(* Logix 5000 AddOnInstructionDefinition export EH_Dosimag_IOL; software revision 38.00 *)

TYPE EH_CommAOI_Data :
STRUCT
   Device_Comm_Error : BOOL;
   CommSuccess : BOOL;
   CommFailed : BOOL;
   CommTimeOut : BOOL;
   StateDone : BOOL;
   NewState : BOOL;
   OldState : SINT;
   PortSize : SINT;
   DevicePort : SINT;
   MaxState : SINT;
   State : SINT;
   VendorID : INT;
   DeviceID : DINT;
   CyclicData : INT[16];
   AcyclicData : DINT[8];
   ReplayIndex : INT;
   AOI_Diagnostic : DINT;
   ConnectionStatus : DINT;
   OutputData : INT[16];
END_STRUCT
END_TYPE

ADD_ON_INSTRUCTION EH_Dosimag_IOL   (* revision 1.1, vendor Endress+Hauser *)
// Dosimag D5AB Rev 1 IO-Link
// Revision note:
// 1.1 Changed the Datatype from Unsigned to Signed
// ZeroPoint adjustment update
// Add Disconnect check
// Add condition PulseSimulation
VAR_IN_OUT
   DataToSend : INT[10]; {required}
   CommAOIBusy : DINT; {required}
   ActiveComPort : DINT; {required}
   DeviceAOISendRequest : DINT; {required}
   CommError : INT; {required}
   DeviceData : EH_CommAOI_Data; {required}
END_VAR
VAR_INPUT
   iSetPulseSimulation : BOOL; {visible}
   iSimulationOnOff : BOOL; {access None, visible}
   iAmountPulses : INT; {visible}
   iSetTotalizerPresetValue : BOOL; {visible}
   iTotalizer1PresetValue : REAL; {visible}
   iTotalizer_Hold : BOOL; {visible}
   iTotalizer_ResetTotalize : BOOL; {visible}
   iTotalizer_ResetHold : BOOL; {visible}
   iTotalizer_Totalize : BOOL; {visible}
   iParameterize : BOOL; {visible}
   iFlowDamping : REAL; {visible}
   iPressureShockSupression : REAL; {visible}
   iIntegrationTime : REAL; {visible}
   iMeasuringPeriod : REAL; {visible}
   iLowFlowCutoffValue : REAL; {visible}
   iFlowOverride : BOOL; {visible}
   iStartZeroPointAdjustment : BOOL; {visible}
END_VAR
VAR_OUTPUT
   qVendor_ID : DINT; {access Read Only, visible}
   qDevice_ID : DINT; {access Read Only, visible}
   qVolumeFlow : REAL; {visible}
   qTemperature : REAL; {visible}
   qTotalizer1 : REAL; {access Read Only, visible}
   qExtendedDeviceStatus : INT; {access Read Only, visible}
   qZeroPointStatus : SINT; {access Read Only, visible}
   qReadProgress : SINT; {access Read Only, visible}
   qSSC1_1 : BOOL; {access Read Only, visible}
   qSSC1_2 : BOOL; {access Read Only, visible}
   qSSC2_1 : BOOL; {access Read Only, visible}
   qSSC2_2 : BOOL; {access Read Only, visible}
   qSSC3_1 : BOOL; {access Read Only, visible}
   qSSC3_2 : BOOL; {access Read Only, visible}
   qSSC4_1 : BOOL; {access Read Only, visible}
   qSSC4_2 : BOOL; {access Read Only, visible}
   qAOI_Diagnostic : DINT; {access Read Only, visible}
END_VAR
VAR_IN_OUT
   qAOI_Diagnostic_String : STRING; {required}
END_VAR
VAR_OUTPUT
   qActual_Diagnostics_Code : DINT; {access Read Only, visible}
END_VAR
VAR_IN_OUT
   qActual_Diagnostics_String : STRING; {required}
END_VAR
VAR_OUTPUT
   qLast_Diagnostics_Code : DINT; {visible}
END_VAR
VAR_IN_OUT
   qLast_Diagnostics_String : STRING; {required}
END_VAR
VAR_OUTPUT
   qCommError : DINT; {access None}
   qCommunicationBusy : DINT; {access Read Only, visible}
   qDeviceConnectionError : BOOL; {access Read Only, visible}
END_VAR
VAR
   Temp_DINT : DINT; {access None}
   CMD_Index : INT; {access None}
   CMD_Subindex : INT; {access None}
   CMD_ByteLength : INT; {access None}
   oldCondStatus : INT; {access None}
   SetSimulation : SINT; {access None}
   SetTotalizer : SINT; {access None}
   oldSetTotalizer : SINT; {access None}
   oldStartZeroPointAdjustment : SINT; {access None}
   Trigger : BOOL; {access None}
   CMD_Rd : BOOL; {access None}
   CMD_Wr : BOOL; {access None}
   SimulationDINT : DINT; {access None}
   AOI_Prio : BOOL; {access None}
   StateMin : DINT; {access None}
   firstTimeDone : BOOL; {access None}
   CondStatusChanged : BOOL; {access None}
   Calc_MassFlow : DINT; {access None}
   Calc_Temperature : DINT; {access None}
   Calc_Totalizer1 : DINT; {access None}
   Calc_ExtendedDeviceStatus : DINT; {access None}
   CondStatusActive : BOOL; {access None}
   ActiveAOI : BOOL; {access None}
   TotActive : BOOL; {access None}
   Skip : BOOL; {access None}
   StartZeroPointAdjustment : SINT; {access None}
   Parameterize : SINT; {access None}
   oldParameterize : SINT; {access None}
   oldSetPulseSimulation : SINT; {access None}
   TotChanged : BOOL; {access None}
   DeviceID : DINT; {access None}
   SetPulseSimulation : SINT; {access None}
   zeroPointStatus : SINT; {access None}
   StartZeroPointAdjustmentChanged : BOOL; {access None}
   ParameterizeChanged : BOOL; {access None}
   PulseSimChanged : BOOL; {access None}
   TRUE : BOOL := 1; {access None}
   FALSE : BOOL; {access None}
   ParameterizeActive : BOOL; {access None}
   PulseSimActive : BOOL; {access None}
   ZeroPointActive : BOOL; {access None}
   StandardTimer : FBD_TIMER; {access None}
   temp_string1 : STRING; {access None}
   temp_string2 : STRING; {access None}
   Calc_VolumeFLow : DINT; {access None}
   IntegrationTimeREAL : REAL; {access None}
   MeasuringPeriodREAL : REAL; {access None}
   onlyonce : BOOL; {access None}
END_VAR

ROUTINE Logic   (* structured text *)
// Picomag Communication via AL1323
   // =======================================================================
   // Endress+Hauser Digital Solutions
   // ©Copyright (2024) All Rights Reserved
   // =======================================================================
   // Name:                EH_Dosimag_IOL
   // Version:             1.1
   // Datum:               02.2026
   // Library:             01.01.00
   // Engineering:         Studio5000 V38.00.00
   // Author:              EH
   // =======================================================================
   
   qAOI_Diagnostic := DeviceData.AOI_Diagnostic;
   qCommunicationBusy := CommAOIBusy;
   DeviceID := 9729281;
   StateMin := 0;
   DeviceData.MaxState := 98;
   
   if DeviceData.DevicePort = 0 or DeviceData.DeviceID <> DeviceID or DeviceData.ConnectionStatus <> 1 then
   
   	qVendor_ID := DeviceData.VendorID;
   	qDevice_ID := DeviceData.DeviceID;
   	qVolumeFlow := 0;
   	qTemperature := 0;
   	qTotalizer1	:= 0;
   	qExtendedDeviceStatus := 0;
   	qSSC1_1	:= FALSE;
   	qSSC1_2	:= FALSE;
   	qSSC2_1	:= FALSE;
   	qSSC2_2	:= FALSE;
   	qSSC3_1	:= FALSE;
   	qSSC3_2	:= FALSE;
   	qSSC4_1	:= FALSE;
   	qSSC4_2	:= FALSE;
   	qActual_Diagnostics_Code := 0;
   	qActual_Diagnostics_String := '';
   	qLast_Diagnostics_Code := 0;
   	qLast_Diagnostics_String := '';
   	qReadProgress := 0;
   	qZeroPointStatus := 0;
   	oldCondStatus := 0;
   	CondStatusChanged := FALSE;
   	zeroPointStatus := 0;
   
   	if DeviceData.DevicePort = 0 then
   
   		qAOI_Diagnostic_String	:= 'Device Port is Zero';
   		DeviceData.AOI_Diagnostic.1 := TRUE;
   
   	elsif DeviceData.ConnectionStatus <> 1 then
   
   		qAOI_Diagnostic_String	:= 'No Device connected';
   		qDeviceConnectionError := TRUE;
   
   	elsif DeviceData.DeviceID <> DeviceID then
   
   		qAOI_Diagnostic_String	:= 'Wrong DeviceID';
   		DeviceData.AOI_Diagnostic.2 := TRUE;
   	end_if;
   
   else
   
   	if qActual_Diagnostics_Code = 0  then
   
   		qActual_Diagnostics_String	:= '--------';
   
   	end_if;
   
   	if qLast_Diagnostics_Code = 0 then
   
   		qLast_Diagnostics_String	:= '--------';
   
   	end_if;
   
   	qAOI_Diagnostic_String := '';
   	DeviceData.AOI_Diagnostic.1 := FALSE;
   	qDeviceConnectionError := FALSE;
   	DeviceData.AOI_Diagnostic.2  := FALSE;
   
   end_if;
   
   // Case device disconnected during communication to avoid blocking the communication
   if (DeviceData.AOI_Diagnostic.0 or qDeviceConnectionError or DeviceData.AOI_Diagnostic.2) and ActiveAOI and ActiveComPort = DeviceData.DevicePort and CommAOIBusy = 1 then
   
   	DeviceData.State := 0;
   	CommAOIBusy := 0;
   	DeviceAOISendRequest.[DeviceData.DevicePort] := 0;
   	ActiveComPort := 0;
   	ActiveAOI := 0;
   	DataToSend[0] := 0;
   	DataToSend[1] := 0;
   	DataToSend[2] := 0;
   	DataToSend[3] := 0;
   	DataToSend[4] := 0;
   	DataToSend[5] := 0;
   	DataToSend[6] := 0;
   	DataToSend[7] := 0;
   	DataToSend[8] := 0;
   	DataToSend[9] := 0;
   	DeviceData.StateDone := FALSE;
   	DeviceData.NewState := FALSE;
   	DeviceData.OldState := 0;
   	ActiveAOI := FALSE;
   
   end_if;
   
   if not DeviceData.AOI_Diagnostic.0
   	and not qDeviceConnectionError
   	and not DeviceData.AOI_Diagnostic.2
   	and DeviceData.DevicePort > 0 then
   
   	//*********************************
   	//Vendor ID
   	//*********************************
   
   		qVendor_ID := DeviceData.VendorID;
   
   	//*********************************
   	//Device ID
   	//*********************************
   
   		qDevice_ID := DeviceData.DeviceID;
   
   	//*********************************
   	// Dosimag
   	//*********************************
   
   		Calc_VolumeFLow			    := 0;
   		// Offset +2 is not used
   		Calc_Temperature			:= 4;
   		Calc_Totalizer1				:= 6;
   		Calc_ExtendedDeviceStatus	:= 8;
   
   	//*********************************
   	//Process VolumeFlow
   	//*********************************
   
   		Temp_DINT	 := DeviceData.CyclicData[Calc_VolumeFLow+1];
   		Temp_DINT.8	 := DeviceData.CyclicData[Calc_VolumeFLow+1].8;
   		Temp_DINT.9  := DeviceData.CyclicData[Calc_VolumeFLow+1].9;
   		Temp_DINT.10 := DeviceData.CyclicData[Calc_VolumeFLow+1].10;
   		Temp_DINT.11 := DeviceData.CyclicData[Calc_VolumeFLow+1].11;
   		Temp_DINT.12 := DeviceData.CyclicData[Calc_VolumeFLow+1].12;
   		Temp_DINT.13 := DeviceData.CyclicData[Calc_VolumeFLow+1].13;
   		Temp_DINT.14 := DeviceData.CyclicData[Calc_VolumeFLow+1].14;
   		Temp_DINT.15 := DeviceData.CyclicData[Calc_VolumeFLow+1].15;
   		Temp_DINT.16 := DeviceData.CyclicData[Calc_VolumeFLow].0;
   		Temp_DINT.17 := DeviceData.CyclicData[Calc_VolumeFLow].1;
   		Temp_DINT.18 := DeviceData.CyclicData[Calc_VolumeFLow].2;
   		Temp_DINT.19 := DeviceData.CyclicData[Calc_VolumeFLow].3;
   		Temp_DINT.20 := DeviceData.CyclicData[Calc_VolumeFLow].4;
   		Temp_DINT.21 := DeviceData.CyclicData[Calc_VolumeFLow].5;
   		Temp_DINT.22 := DeviceData.CyclicData[Calc_VolumeFLow].6;
   		Temp_DINT.23 := DeviceData.CyclicData[Calc_VolumeFLow].7;
   		Temp_DINT.24 := DeviceData.CyclicData[Calc_VolumeFLow].8;
   		Temp_DINT.25 := DeviceData.CyclicData[Calc_VolumeFLow].9;
   		Temp_DINT.26 := DeviceData.CyclicData[Calc_VolumeFLow].10;
   		Temp_DINT.27 := DeviceData.CyclicData[Calc_VolumeFLow].11;
   		Temp_DINT.28 := DeviceData.CyclicData[Calc_VolumeFLow].12;
   		Temp_DINT.29 := DeviceData.CyclicData[Calc_VolumeFLow].13;
   		Temp_DINT.30 := DeviceData.CyclicData[Calc_VolumeFLow].14;
   		Temp_DINT.31 := DeviceData.CyclicData[Calc_VolumeFLow].15;
   
   		COP(Temp_DINT,qVolumeFlow,1);
   
   
   	//*********************************
   	//Process Data Temperature
   	//*********************************
   
   		Temp_DINT	 := DeviceData.CyclicData[Calc_Temperature+1];
   		Temp_DINT.8	 := DeviceData.CyclicData[Calc_Temperature+1].8;
   		Temp_DINT.9	 := DeviceData.CyclicData[Calc_Temperature+1].9;
   		Temp_DINT.10 := DeviceData.CyclicData[Calc_Temperature+1].10;
   		Temp_DINT.11 := DeviceData.CyclicData[Calc_Temperature+1].11;
   		Temp_DINT.12 := DeviceData.CyclicData[Calc_Temperature+1].12;
   		Temp_DINT.13 := DeviceData.CyclicData[Calc_Temperature+1].13;
   		Temp_DINT.14 := DeviceData.CyclicData[Calc_Temperature+1].14;
   		Temp_DINT.15 := DeviceData.CyclicData[Calc_Temperature+1].15;
   		Temp_DINT.16 := DeviceData.CyclicData[Calc_Temperature].0;
   		Temp_DINT.17 := DeviceData.CyclicData[Calc_Temperature].1;
   		Temp_DINT.18 := DeviceData.CyclicData[Calc_Temperature].2;
   		Temp_DINT.19 := DeviceData.CyclicData[Calc_Temperature].3;
   		Temp_DINT.20 := DeviceData.CyclicData[Calc_Temperature].4;
   		Temp_DINT.21 := DeviceData.CyclicData[Calc_Temperature].5;
   		Temp_DINT.22 := DeviceData.CyclicData[Calc_Temperature].6;
   		Temp_DINT.23 := DeviceData.CyclicData[Calc_Temperature].7;
   		Temp_DINT.24 := DeviceData.CyclicData[Calc_Temperature].8;
   		Temp_DINT.25 := DeviceData.CyclicData[Calc_Temperature].9;
   		Temp_DINT.26 := DeviceData.CyclicData[Calc_Temperature].10;
   		Temp_DINT.27 := DeviceData.CyclicData[Calc_Temperature].11;
   		Temp_DINT.28 := DeviceData.CyclicData[Calc_Temperature].12;
   		Temp_DINT.29 := DeviceData.CyclicData[Calc_Temperature].13;
   		Temp_DINT.30 := DeviceData.CyclicData[Calc_Temperature].14;
   		Temp_DINT.31 := DeviceData.CyclicData[Calc_Temperature].15;
   
   		COP(Temp_DINT,qTemperature,1);
   
   	//*********************************
   	// Process Parameter Totalizer1
   	//*********************************
   
   		Temp_DINT	 := DeviceData.CyclicData[Calc_Totalizer1+1];
   		Temp_DINT.8  := DeviceData.CyclicData[Calc_Totalizer1+1].8;
   		Temp_DINT.9  := DeviceData.CyclicData[Calc_Totalizer1+1].9;
   		Temp_DINT.10 := DeviceData.CyclicData[Calc_Totalizer1+1].10;
   		Temp_DINT.11 := DeviceData.CyclicData[Calc_Totalizer1+1].11;
   		Temp_DINT.12 := DeviceData.CyclicData[Calc_Totalizer1+1].12;
   		Temp_DINT.13 := DeviceData.CyclicData[Calc_Totalizer1+1].13;
   		Temp_DINT.14 := DeviceData.CyclicData[Calc_Totalizer1+1].14;
   		Temp_DINT.15 := DeviceData.CyclicData[Calc_Totalizer1+1].15;
   		Temp_DINT.16 := DeviceData.CyclicData[Calc_Totalizer1].0;
   		Temp_DINT.17 := DeviceData.CyclicData[Calc_Totalizer1].1;
   		Temp_DINT.18 := DeviceData.CyclicData[Calc_Totalizer1].2;
   		Temp_DINT.19 := DeviceData.CyclicData[Calc_Totalizer1].3;
   		Temp_DINT.20 := DeviceData.CyclicData[Calc_Totalizer1].4;
   		Temp_DINT.21 := DeviceData.CyclicData[Calc_Totalizer1].5;
   		Temp_DINT.22 := DeviceData.CyclicData[Calc_Totalizer1].6;
   		Temp_DINT.23 := DeviceData.CyclicData[Calc_Totalizer1].7;
   		Temp_DINT.24 := DeviceData.CyclicData[Calc_Totalizer1].8;
   		Temp_DINT.25 := DeviceData.CyclicData[Calc_Totalizer1].9;
   		Temp_DINT.26 := DeviceData.CyclicData[Calc_Totalizer1].10;
   		Temp_DINT.27 := DeviceData.CyclicData[Calc_Totalizer1].11;
   		Temp_DINT.28 := DeviceData.CyclicData[Calc_Totalizer1].12;
   		Temp_DINT.29 := DeviceData.CyclicData[Calc_Totalizer1].13;
   		Temp_DINT.30 := DeviceData.CyclicData[Calc_Totalizer1].14;
   		Temp_DINT.31 := DeviceData.CyclicData[Calc_Totalizer1].15;
   
   		COP(Temp_DINT,qTotalizer1,1);
   
   	//*********************************
   	// Extended device Status
   	//*********************************
   
   		qExtendedDeviceStatus.0 := DeviceData.CyclicData[Calc_ExtendedDeviceStatus].8;
   		qExtendedDeviceStatus.1 := DeviceData.CyclicData[Calc_ExtendedDeviceStatus].9;
   		qExtendedDeviceStatus.2 := DeviceData.CyclicData[Calc_ExtendedDeviceStatus].10;
   		qExtendedDeviceStatus.3 := DeviceData.CyclicData[Calc_ExtendedDeviceStatus].11;
   		qExtendedDeviceStatus.4 := DeviceData.CyclicData[Calc_ExtendedDeviceStatus].12;
   		qExtendedDeviceStatus.5 := DeviceData.CyclicData[Calc_ExtendedDeviceStatus].13;
   		qExtendedDeviceStatus.6 := DeviceData.CyclicData[Calc_ExtendedDeviceStatus].14;
   		qExtendedDeviceStatus.7 := DeviceData.CyclicData[Calc_ExtendedDeviceStatus].15;
   
   	//*********************************
   	// Process Parameter SSC
   	//*********************************
   
   		qSSC1_1 := DeviceData.CyclicData[Calc_ExtendedDeviceStatus].0;
   		qSSC1_2 := DeviceData.CyclicData[Calc_ExtendedDeviceStatus].1;
   
   		qSSC2_1 := DeviceData.CyclicData[Calc_ExtendedDeviceStatus].2;
   		qSSC2_2 := DeviceData.CyclicData[Calc_ExtendedDeviceStatus].3;
   
   		qSSC3_1 := DeviceData.CyclicData[Calc_ExtendedDeviceStatus].4;
   		qSSC3_2 := DeviceData.CyclicData[Calc_ExtendedDeviceStatus].5;
   
   		qSSC4_1 := DeviceData.CyclicData[Calc_ExtendedDeviceStatus].6;
   		qSSC4_2 := DeviceData.CyclicData[Calc_ExtendedDeviceStatus].7;
   
   	//*********************************
   	// Process Output Parameter
   	//*********************************
   
   		//DeviceData.OutputData[0].4 := iDeviceSearch;		//Device Specific
   		DeviceData.OutputData[0].5 := iFlowOverride;
   		DeviceData.OutputData[0].6 := iTotalizer_Hold;
   		DeviceData.OutputData[0].7 := iTotalizer_ResetTotalize;
   		DeviceData.OutputData[0].8 := iTotalizer_ResetHold;
   		DeviceData.OutputData[0].9 := iTotalizer_Totalize;
   
   	//*********************************
   	// Checking for Changed Status
   	//*********************************
   
   		SetPulseSimulation.0 := iSetPulseSimulation;
   		SetTotalizer.0 := iSetTotalizerPresetValue;
   		Parameterize.0 := iParameterize;
   		StartZeroPointAdjustment.0 := iStartZeroPointAdjustment;
   
   		if oldCondStatus <> qExtendedDeviceStatus and not CondStatusChanged then
   
   			CondStatusChanged := TRUE;
   			oldCondStatus := qExtendedDeviceStatus;
   
   		end_if;
   
   		if oldSetPulseSimulation <> SetPulseSimulation and not PulseSimChanged then
   
   			if oldSetPulseSimulation < SetPulseSimulation then
   
   				PulseSimChanged := TRUE;
   
   			end_if;
   
   			oldSetPulseSimulation := SetPulseSimulation;
   
   		end_if;
   
   		if oldStartZeroPointAdjustment <> StartZeroPointAdjustment and not StartZeroPointAdjustmentChanged then
   
   			if oldStartZeroPointAdjustment < StartZeroPointAdjustment then
   
   				StartZeroPointAdjustmentChanged := TRUE;
   
   			end_if;
   
   			oldStartZeroPointAdjustment := StartZeroPointAdjustment;
   
   		end_if;
   
   		if oldParameterize <> Parameterize and not ParameterizeChanged then
   
   			if oldParameterize < Parameterize then
   
   				ParameterizeChanged := TRUE;
   
   			end_if;
   
   			oldParameterize := Parameterize;
   
   		end_if;
   
   		if oldSetTotalizer <> SetTotalizer and not TotChanged then
   
   			if oldSetTotalizer < SetTotalizer then
   
   				TotChanged := TRUE;
   
   			end_if;
   
   			oldSetTotalizer := SetTotalizer;
   
   		end_if;
   
   		if CondStatusChanged
   		and not ActiveAOI
   		and not CondStatusActive
   		and not Skip then
   
   			DeviceAOISendRequest.[DeviceData.DevicePort] := TRUE;
   			CondStatusActive := TRUE;
   			Skip := TRUE;
   
   		elsif PulseSimChanged
   			and not ActiveAOI
   			and not PulseSimActive
   			and not Skip then
   
   			DeviceAOISendRequest.[DeviceData.DevicePort] := TRUE;
   			PulseSimActive := TRUE;
   			Skip := TRUE;
   
   		elsif TotChanged
   			and not ActiveAOI
   			and not TotActive
   			and not Skip then
   
   			DeviceAOISendRequest.[DeviceData.DevicePort] := TRUE;
   			TotActive := TRUE;
   			Skip := TRUE;
   
   		elsif StartZeroPointAdjustmentChanged
   			and not ActiveAOI
   			and not ZeroPointActive
   			and not Skip then
   
   			DeviceAOISendRequest.[DeviceData.DevicePort] := TRUE;
   			ZeroPointActive := TRUE;
   			Skip := TRUE;
   
   		elsif ParameterizeChanged
   			and not ActiveAOI
   			and not ParameterizeActive
   			and not Skip then
   
   			DeviceAOISendRequest.[DeviceData.DevicePort] := TRUE;
   			ParameterizeActive := TRUE;
   			Skip := TRUE;
   
   		end_if;
   
   		if ActiveComPort = DeviceData.DevicePort then
   
   			AOI_Prio :=TRUE;
   
   		else
   
   			AOI_Prio := FALSE;
   
   		end_if;
   
   		if (PulseSimActive or TotActive or CondStatusActive or ParameterizeActive or ZeroPointActive) and CommAOIBusy = 1  and DeviceData.State = 0 and AOI_Prio and not ActiveAOI then
   
   			ActiveAOI := TRUE;
   			Skip := FALSE;
   
   		end_if;
   
   		qCommunicationBusy := CommAOIBusy;
   		qAOI_Diagnostic :=DeviceData.AOI_Diagnostic;
   
   	//*********************************
   	// States for Execution
   	//*********************************
   
   	if ActiveAOI or DeviceData.State = DeviceData.MaxState then
   
   	case DeviceData.State of
   
   		//*********************************
   		0: // Idle
   		//*********************************
   
   			// Initializing
   			Trigger := FALSE;
   			CMD_Index := 0;
   			CMD_Subindex := 0;
   			CMD_Wr := FALSE;
   			CMD_Rd := FALSE;
   		    CMD_ByteLength := 0;
   
   			if DeviceData.DevicePort = ActiveComPort then
   					DeviceData.CommSuccess := FALSE;
   					DeviceData.CommTimeOut := FALSE;
   					DeviceData.NewState := TRUE;
   					DeviceData.StateDone := FALSE;
   			end_if;
   
   			// Wait for trigger
   			if ParameterizeActive then
   
   				DeviceData.AOI_Diagnostic := 0;
   				DeviceData.State := 6;
   
   			elsif PulseSimActive then
   
   				DeviceData.AOI_Diagnostic := 0;
   				DeviceData.State := 15;
   
   			elsif TotActive then
   				DeviceData.AOI_Diagnostic := 0;
   				DeviceData.State := 20;
   
   			elsif ZeroPointActive then
   
   				DeviceData.AOI_Diagnostic := 0;
   				qReadProgress := 0;
   				qZeroPointStatus := 0;
   				DeviceData.State := 30;
   
   			elsif CondStatusChanged then
   
   				DeviceData.State := 90;
   
   			end_if;
   
   		//*********************************
   		6: // Set Flow Damping
   		//*********************************
   
   			CMD_Index := 8550;
   			CMD_Subindex := 0;
   			CMD_Wr := TRUE;
   			CMD_Rd := FALSE;
   			CMD_ByteLength := 4;
   			DataToSend[6]:= 0;
   			DataToSend[7]:= 0;
   
   			// Time in seconds
   			COP(iFlowDamping,SimulationDINT,1);		// Copy the Bits from the Real in a DINT
   
   			DataToSend[6].0 :=  SimulationDINT.24;
   			DataToSend[6].1 :=  SimulationDINT.25;
   			DataToSend[6].2 :=  SimulationDINT.26;
   			DataToSend[6].3 :=  SimulationDINT.27;
   			DataToSend[6].4 :=  SimulationDINT.28;
   			DataToSend[6].5 :=  SimulationDINT.29;
   			DataToSend[6].6 :=  SimulationDINT.30;
   			DataToSend[6].7 :=  SimulationDINT.31;
   			DataToSend[6].8 :=  SimulationDINT.16;
   			DataToSend[6].9 :=  SimulationDINT.17;
   			DataToSend[6].10 := SimulationDINT.18;
   			DataToSend[6].11 := SimulationDINT.19;
   			DataToSend[6].12 := SimulationDINT.20;
   			DataToSend[6].13 := SimulationDINT.21;
   			DataToSend[6].14 := SimulationDINT.22;
   			DataToSend[6].15 := SimulationDINT.23;
   			DataToSend[7].0  := SimulationDINT.8;
   			DataToSend[7].1  := SimulationDINT.9;
   			DataToSend[7].2  := SimulationDINT.10;
   			DataToSend[7].3  := SimulationDINT.11;
   			DataToSend[7].4  := SimulationDINT.12;
   			DataToSend[7].5  := SimulationDINT.13;
   			DataToSend[7].6  := SimulationDINT.14;
   			DataToSend[7].7  := SimulationDINT.15;
   			DataToSend[7].8  := SimulationDINT.0;
   			DataToSend[7].9  := SimulationDINT.1;
   			DataToSend[7].10 := SimulationDINT.2;
   			DataToSend[7].11 := SimulationDINT.3;
   			DataToSend[7].12 := SimulationDINT.4;
   			DataToSend[7].13 := SimulationDINT.5;
   			DataToSend[7].14 := SimulationDINT.6;
   			DataToSend[7].15 := SimulationDINT.7;
   
   			Trigger := TRUE;
   
   			if DeviceData.NewState then
   
   				DeviceData.StateDone := TRUE;
   
   			end_if;
   
   			if DeviceData.CommSuccess and DeviceData.ReplayIndex = CMD_Index then
   
   				Trigger := FALSE;
   				DeviceData.OldState := DeviceData.State;
   				DeviceData.State := DeviceData.State + 1;
   				DeviceData.CommSuccess := FALSE;
   				DeviceData.AcyclicData[0] := 0;
   				DeviceData.NewState := TRUE;
   
   			elsif DeviceData.CommTimeOut then
   
   				temp_string1 := 'Error in step ';
   				Temp_DINT := DeviceData.State;
   				DTOS(Temp_DINT, temp_string2);
   				CONCAT(temp_string1, temp_string2, qAOI_Diagnostic_String);
   
   				DeviceData.OldState := DeviceData.State;
   				DeviceData.State := DeviceData.MaxState;	//Check State
   				DeviceData.CommTimeOut := FALSE;
   				DeviceData.AcyclicData[0] := 0;
   				DeviceData.NewState := TRUE;
   
   			end_if;
   
   		//*********************************
   		7: // Set pressure shock supression
   		//*********************************
   
   			CMD_Index := 2108;
   			CMD_Subindex := 0;
   			CMD_Wr := TRUE;
   			CMD_Rd := FALSE;
   			CMD_ByteLength := 4;
   			DataToSend[6]:= 0;
   			DataToSend[7]:= 0;
   
   			// Time in seconds
   			COP(iPressureShockSupression,SimulationDINT,1);		// Copy the Bits from the Real in a DINT
   
   			DataToSend[6].0 :=  SimulationDINT.24;
   			DataToSend[6].1 :=  SimulationDINT.25;
   			DataToSend[6].2 :=  SimulationDINT.26;
   			DataToSend[6].3 :=  SimulationDINT.27;
   			DataToSend[6].4 :=  SimulationDINT.28;
   			DataToSend[6].5 :=  SimulationDINT.29;
   			DataToSend[6].6 :=  SimulationDINT.30;
   			DataToSend[6].7 :=  SimulationDINT.31;
   			DataToSend[6].8 :=  SimulationDINT.16;
   			DataToSend[6].9 :=  SimulationDINT.17;
   			DataToSend[6].10 := SimulationDINT.18;
   			DataToSend[6].11 := SimulationDINT.19;
   			DataToSend[6].12 := SimulationDINT.20;
   			DataToSend[6].13 := SimulationDINT.21;
   			DataToSend[6].14 := SimulationDINT.22;
   			DataToSend[6].15 := SimulationDINT.23;
   			DataToSend[7].0  := SimulationDINT.8;
   			DataToSend[7].1  := SimulationDINT.9;
   			DataToSend[7].2  := SimulationDINT.10;
   			DataToSend[7].3  := SimulationDINT.11;
   			DataToSend[7].4  := SimulationDINT.12;
   			DataToSend[7].5  := SimulationDINT.13;
   			DataToSend[7].6  := SimulationDINT.14;
   			DataToSend[7].7  := SimulationDINT.15;
   			DataToSend[7].8  := SimulationDINT.0;
   			DataToSend[7].9  := SimulationDINT.1;
   			DataToSend[7].10 := SimulationDINT.2;
   			DataToSend[7].11 := SimulationDINT.3;
   			DataToSend[7].12 := SimulationDINT.4;
   			DataToSend[7].13 := SimulationDINT.5;
   			DataToSend[7].14 := SimulationDINT.6;
   			DataToSend[7].15 := SimulationDINT.7;
   
   			Trigger := TRUE;
   
   			if DeviceData.NewState then
   
   				DeviceData.StateDone := TRUE;
   
   			end_if;
   
   			if DeviceData.CommSuccess and DeviceData.ReplayIndex = CMD_Index then
   
   				Trigger := FALSE;
   				DeviceData.OldState := DeviceData.State;
   				DeviceData.State := DeviceData.State + 1;
   				DeviceData.CommSuccess := FALSE;
   				DeviceData.AcyclicData[0] := 0;
   				DeviceData.NewState := TRUE;
   
   			elsif DeviceData.CommTimeOut then
   
   				temp_string1 := 'Error in step ';
   				Temp_DINT := DeviceData.State;
   				DTOS(Temp_DINT, temp_string2);
   				CONCAT(temp_string1, temp_string2, qAOI_Diagnostic_String);
   
   				DeviceData.OldState := DeviceData.State;
   				DeviceData.State := DeviceData.MaxState;	//Check State
   				DeviceData.CommTimeOut := FALSE;
   				DeviceData.AcyclicData[0] := 0;
   				DeviceData.NewState := TRUE;
   
   			end_if;
   
   		//*********************************
   		8: // Integration Time
   		//*********************************
   
   			CMD_Index := 8600;
   			CMD_Subindex := 0;
   			CMD_Wr := TRUE;
   			CMD_Rd := FALSE;
   			CMD_ByteLength := 4;
   			DataToSend[6]:= 0;
   			DataToSend[7]:= 0;
   
   			// Time in seconds
   			if iIntegrationTime < 0.001 or iIntegrationTime > 0.065 then
   				IntegrationTimeREAL := 0.005; // Default value in IODD
   			else
   				IntegrationTimeREAL := iIntegrationTime;
   			end_if;
   
   			COP(IntegrationTimeREAL,SimulationDINT,1);		// Copy the Bits from the Real in a DINT
   
   			DataToSend[6].0 :=  SimulationDINT.24;
   			DataToSend[6].1 :=  SimulationDINT.25;
   			DataToSend[6].2 :=  SimulationDINT.26;
   			DataToSend[6].3 :=  SimulationDINT.27;
   			DataToSend[6].4 :=  SimulationDINT.28;
   			DataToSend[6].5 :=  SimulationDINT.29;
   			DataToSend[6].6 :=  SimulationDINT.30;
   			DataToSend[6].7 :=  SimulationDINT.31;
   			DataToSend[6].8 :=  SimulationDINT.16;
   			DataToSend[6].9 :=  SimulationDINT.17;
   			DataToSend[6].10 := SimulationDINT.18;
   			DataToSend[6].11 := SimulationDINT.19;
   			DataToSend[6].12 := SimulationDINT.20;
   			DataToSend[6].13 := SimulationDINT.21;
   			DataToSend[6].14 := SimulationDINT.22;
   			DataToSend[6].15 := SimulationDINT.23;
   			DataToSend[7].0  := SimulationDINT.8;
   			DataToSend[7].1  := SimulationDINT.9;
   			DataToSend[7].2  := SimulationDINT.10;
   			DataToSend[7].3  := SimulationDINT.11;
   			DataToSend[7].4  := SimulationDINT.12;
   			DataToSend[7].5  := SimulationDINT.13;
   			DataToSend[7].6  := SimulationDINT.14;
   			DataToSend[7].7  := SimulationDINT.15;
   			DataToSend[7].8  := SimulationDINT.0;
   			DataToSend[7].9  := SimulationDINT.1;
   			DataToSend[7].10 := SimulationDINT.2;
   			DataToSend[7].11 := SimulationDINT.3;
   			DataToSend[7].12 := SimulationDINT.4;
   			DataToSend[7].13 := SimulationDINT.5;
   			DataToSend[7].14 := SimulationDINT.6;
   			DataToSend[7].15 := SimulationDINT.7;
   
   			Trigger := TRUE;
   
   			if DeviceData.NewState then
   
   				DeviceData.StateDone := TRUE;
   
   			end_if;
   
   			if DeviceData.CommSuccess and DeviceData.ReplayIndex = CMD_Index then
   
   				Trigger := FALSE;
   				DeviceData.OldState := DeviceData.State;
   				DeviceData.State := DeviceData.State + 1;
   				DeviceData.CommSuccess := FALSE;
   				DeviceData.AcyclicData[0] := 0;
   				DeviceData.NewState := TRUE;
   
   			elsif DeviceData.CommTimeOut then
   
   				temp_string1 := 'Error in step ';
   				Temp_DINT := DeviceData.State;
   				DTOS(Temp_DINT, temp_string2);
   				CONCAT(temp_string1, temp_string2, qAOI_Diagnostic_String);
   
   				DeviceData.OldState := DeviceData.State;
   				DeviceData.State := DeviceData.MaxState;	//Check State
   				DeviceData.CommTimeOut := FALSE;
   				DeviceData.AcyclicData[0] := 0;
   				DeviceData.NewState := TRUE;
   
   			end_if;
   
   		//*********************************
   		9: // Measuring period
   		//*********************************
   
   			CMD_Index := 8599;
   			CMD_Subindex := 0;
   			CMD_Wr := TRUE;
   			CMD_Rd := FALSE;
   			CMD_ByteLength := 4;
   			DataToSend[6]:= 0;
   			DataToSend[7]:= 0;
   
   			// Time in seconds
   			if iMeasuringPeriod < 0.0 or iMeasuringPeriod > 1.0 then
   				MeasuringPeriodREAL := 0.0125; // Default value in IODD
   			else
   				MeasuringPeriodREAL := iMeasuringPeriod;
   			end_if;
   
   			COP(MeasuringPeriodREAL,SimulationDINT,1);		// Copy the Bits from the Real in a DINT
   
   			DataToSend[6].0 :=  SimulationDINT.24;
   			DataToSend[6].1 :=  SimulationDINT.25;
   			DataToSend[6].2 :=  SimulationDINT.26;
   			DataToSend[6].3 :=  SimulationDINT.27;
   			DataToSend[6].4 :=  SimulationDINT.28;
   			DataToSend[6].5 :=  SimulationDINT.29;
   			DataToSend[6].6 :=  SimulationDINT.30;
   			DataToSend[6].7 :=  SimulationDINT.31;
   			DataToSend[6].8 :=  SimulationDINT.16;
   			DataToSend[6].9 :=  SimulationDINT.17;
   			DataToSend[6].10 := SimulationDINT.18;
   			DataToSend[6].11 := SimulationDINT.19;
   			DataToSend[6].12 := SimulationDINT.20;
   			DataToSend[6].13 := SimulationDINT.21;
   			DataToSend[6].14 := SimulationDINT.22;
   			DataToSend[6].15 := SimulationDINT.23;
   			DataToSend[7].0  := SimulationDINT.8;
   			DataToSend[7].1  := SimulationDINT.9;
   			DataToSend[7].2  := SimulationDINT.10;
   			DataToSend[7].3  := SimulationDINT.11;
   			DataToSend[7].4  := SimulationDINT.12;
   			DataToSend[7].5  := SimulationDINT.13;
   			DataToSend[7].6  := SimulationDINT.14;
   			DataToSend[7].7  := SimulationDINT.15;
   			DataToSend[7].8  := SimulationDINT.0;
   			DataToSend[7].9  := SimulationDINT.1;
   			DataToSend[7].10 := SimulationDINT.2;
   			DataToSend[7].11 := SimulationDINT.3;
   			DataToSend[7].12 := SimulationDINT.4;
   			DataToSend[7].13 := SimulationDINT.5;
   			DataToSend[7].14 := SimulationDINT.6;
   			DataToSend[7].15 := SimulationDINT.7;
   
   			Trigger := TRUE;
   
   			if DeviceData.NewState then
   
   				DeviceData.StateDone := TRUE;
   
   			end_if;
   
   			if DeviceData.CommSuccess and DeviceData.ReplayIndex = CMD_Index then
   
   				Trigger := FALSE;
   				DeviceData.OldState := DeviceData.State;
   				DeviceData.State := DeviceData.State + 1;
   				DeviceData.CommSuccess := FALSE;
   				DeviceData.AcyclicData[0] := 0;
   				DeviceData.NewState := TRUE;
   
   			elsif DeviceData.CommTimeOut then
   
   				temp_string1 := 'Error in step ';
   				Temp_DINT := DeviceData.State;
   				DTOS(Temp_DINT, temp_string2);
   				CONCAT(temp_string1, temp_string2, qAOI_Diagnostic_String);
   
   				DeviceData.OldState := DeviceData.State;
   				DeviceData.State := DeviceData.MaxState;	//Check State
   				DeviceData.CommTimeOut := FALSE;
   				DeviceData.AcyclicData[0] := 0;
   				DeviceData.NewState := TRUE;
   
   			end_if;
   
   		//*********************************
   		10: // Low flow cut off value
   		//*********************************
   
   			CMD_Index := 2067;
   			CMD_Subindex := 0;
   			CMD_Wr := TRUE;
   			CMD_Rd := FALSE;
   			CMD_ByteLength := 4;
   			DataToSend[6]:= 0;
   			DataToSend[7]:= 0;
   
   
   			COP(iLowFlowCutoffValue ,SimulationDINT,1);		// Copy the Bits from the Real in a DINT
   
   			DataToSend[6].0 :=  SimulationDINT.24;
   			DataToSend[6].1 :=  SimulationDINT.25;
   			DataToSend[6].2 :=  SimulationDINT.26;
   			DataToSend[6].3 :=  SimulationDINT.27;
   			DataToSend[6].4 :=  SimulationDINT.28;
   			DataToSend[6].5 :=  SimulationDINT.29;
   			DataToSend[6].6 :=  SimulationDINT.30;
   			DataToSend[6].7 :=  SimulationDINT.31;
   			DataToSend[6].8 :=  SimulationDINT.16;
   			DataToSend[6].9 :=  SimulationDINT.17;
   			DataToSend[6].10 := SimulationDINT.18;
   			DataToSend[6].11 := SimulationDINT.19;
   			DataToSend[6].12 := SimulationDINT.20;
   			DataToSend[6].13 := SimulationDINT.21;
   			DataToSend[6].14 := SimulationDINT.22;
   			DataToSend[6].15 := SimulationDINT.23;
   			DataToSend[7].0  := SimulationDINT.8;
   			DataToSend[7].1  := SimulationDINT.9;
   			DataToSend[7].2  := SimulationDINT.10;
   			DataToSend[7].3  := SimulationDINT.11;
   			DataToSend[7].4  := SimulationDINT.12;
   			DataToSend[7].5  := SimulationDINT.13;
   			DataToSend[7].6  := SimulationDINT.14;
   			DataToSend[7].7  := SimulationDINT.15;
   			DataToSend[7].8  := SimulationDINT.0;
   			DataToSend[7].9  := SimulationDINT.1;
   			DataToSend[7].10 := SimulationDINT.2;
   			DataToSend[7].11 := SimulationDINT.3;
   			DataToSend[7].12 := SimulationDINT.4;
   			DataToSend[7].13 := SimulationDINT.5;
   			DataToSend[7].14 := SimulationDINT.6;
   			DataToSend[7].15 := SimulationDINT.7;
   
   			Trigger := TRUE;
   
   			if DeviceData.NewState then
   
   				DeviceData.StateDone := TRUE;
   
   			end_if;
   
   			if DeviceData.CommSuccess and DeviceData.ReplayIndex = CMD_Index then
   
   				Trigger := FALSE;
   				DeviceData.OldState := DeviceData.State;
   				DeviceData.State := DeviceData.MaxState;
   				DeviceData.CommSuccess := FALSE;
   				DeviceData.AcyclicData[0] := 0;
   				DeviceData.NewState := TRUE;
   
   			elsif DeviceData.CommTimeOut then
   
   				temp_string1 := 'Error in step ';
   				Temp_DINT := DeviceData.State;
   				DTOS(Temp_DINT, temp_string2);
   				CONCAT(temp_string1, temp_string2, qAOI_Diagnostic_String);
   
   				DeviceData.OldState := DeviceData.State;
   				DeviceData.State := DeviceData.MaxState;	//Check State
   				DeviceData.CommTimeOut := FALSE;
   				DeviceData.AcyclicData[0] := 0;
   				DeviceData.NewState := TRUE;
   
   			end_if;
   
   		//***************************************
   		15: // Set pulse simulation to count down
   		//***************************************
   
   			CMD_Index := 372;
   			CMD_Subindex := 0;
   			CMD_Wr := TRUE;								// Only Read or Write can be active = 1
   			CMD_Rd := FALSE;
   			CMD_ByteLength := 2;
   			DataToSend[6] := 0;
   			DataToSend[7] := 0;
   
   			if iSimulationOnOff then
   
   				DataToSend[6].8 := TRUE;
   				DataToSend[7] := 0;
   
   			else
   
   				DataToSend[6] := 0;
   				DataToSend[7] := 0;
   
   			end_if;
   
   			Trigger := TRUE;
   
   			if DeviceData.NewState then
   
   				DeviceData.StateDone := TRUE;
   
   			end_if;
   
   			if  DeviceData.CommSuccess and DeviceData.ReplayIndex = CMD_Index then
   
   				Trigger := FALSE;
   				DeviceData.OldState := DeviceData.State;
   				if iSimulationOnOff then
   					DeviceData.State := DeviceData.State + 1;
   				else
   					DeviceData.State := DeviceData.MaxState;
   				end_if;
   				DeviceData.CommSuccess := FALSE;
   				DeviceData.AcyclicData[0] := 0;
   				DeviceData.NewState := TRUE;
   
   			elsif DeviceData.CommTimeOut then
   
   				temp_string1 := 'Error in step ';
   				Temp_DINT := DeviceData.State;
   				DTOS(Temp_DINT, temp_string2);
   				CONCAT(temp_string1, temp_string2, qAOI_Diagnostic_String);
   
   				DeviceData.OldState := DeviceData.State;
   				DeviceData.State := DeviceData.MaxState;	//Check State
   				DeviceData.CommTimeOut := FALSE;
   				DeviceData.AcyclicData[0] := 0;
   				DeviceData.NewState := TRUE;
   
   			end_if;
   
   
   		//*********************************
   		16: // Set pulse simulation value
   		//*********************************
   
   			CMD_Index := 373;
   			CMD_Subindex := 0;
   			CMD_Wr := TRUE;
   			CMD_Rd := FALSE;
   			CMD_ByteLength := 2;
   			DataToSend[6]:= 0;
   			DataToSend[7]:= 0;
   
   		 	COP(iAmountPulses,SimulationDINT,1);		// Copy the Bits from the Real in a DINT
   
   			DataToSend[6].0 :=  SimulationDINT.8;
   			DataToSend[6].1 :=  SimulationDINT.9;
   			DataToSend[6].2 :=  SimulationDINT.10;
   			DataToSend[6].3 :=  SimulationDINT.11;
   			DataToSend[6].4 :=  SimulationDINT.12;
   			DataToSend[6].5 :=  SimulationDINT.13;
   			DataToSend[6].6 :=  SimulationDINT.14;
   			DataToSend[6].7 :=  SimulationDINT.15;
   			DataToSend[6].8 :=  SimulationDINT.0;
   			DataToSend[6].9 :=  SimulationDINT.1;
   			DataToSend[6].10 := SimulationDINT.2;
   			DataToSend[6].11 := SimulationDINT.3;
   			DataToSend[6].12 := SimulationDINT.4;
   			DataToSend[6].13 := SimulationDINT.5;
   			DataToSend[6].14 := SimulationDINT.6;
   			DataToSend[6].15 := SimulationDINT.7;
   
   			Trigger := TRUE;
   
   			if DeviceData.NewState then
   
   				DeviceData.StateDone := TRUE;
   
   			end_if;
   
   			if DeviceData.CommSuccess and DeviceData.ReplayIndex = CMD_Index then
   
   				Trigger := FALSE;
   				DeviceData.OldState := DeviceData.State;
   				DeviceData.State := DeviceData.MaxState;
   				DeviceData.CommSuccess := FALSE;
   				DeviceData.AcyclicData[0] := 0;
   				DeviceData.NewState := TRUE;
   
   			elsif DeviceData.CommTimeOut then
   
   				temp_string1 := 'Error in step ';
   				Temp_DINT := DeviceData.State;
   				DTOS(Temp_DINT, temp_string2);
   				CONCAT(temp_string1, temp_string2, qAOI_Diagnostic_String);
   
   				DeviceData.OldState := DeviceData.State;
   				DeviceData.State := DeviceData.MaxState;	//Check State
   				DeviceData.CommTimeOut := FALSE;
   				DeviceData.AcyclicData[0] := 0;
   				DeviceData.NewState := TRUE;
   
   			end_if;
   
   		//*********************************
   		20: // Totalizer 1 preset value
   		//*********************************
   
   			CMD_Index := 2103;
   			CMD_Subindex := 0;
   			CMD_Wr := TRUE;								// Only Read or Write can be active = 1
   			CMD_Rd := FALSE;
   			CMD_ByteLength := 4;
   			DataToSend[6]:= 0;
   			DataToSend[7]:= 0;
   
   		 	COP(iTotalizer1PresetValue,SimulationDINT,1); // Copy the Bits from the Real in a DINT
   
   			DataToSend[6].0 :=  SimulationDINT.24;
   			DataToSend[6].1 :=  SimulationDINT.25;
   			DataToSend[6].2 :=  SimulationDINT.26;
   			DataToSend[6].3 :=  SimulationDINT.27;
   			DataToSend[6].4 :=  SimulationDINT.28;
   			DataToSend[6].5 :=  SimulationDINT.29;
   			DataToSend[6].6 :=  SimulationDINT.30;
   			DataToSend[6].7 :=  SimulationDINT.31;
   			DataToSend[6].8 :=  SimulationDINT.16;
   			DataToSend[6].9 :=  SimulationDINT.17;
   			DataToSend[6].10 := SimulationDINT.18;
   			DataToSend[6].11 := SimulationDINT.19;
   			DataToSend[6].12 := SimulationDINT.20;
   			DataToSend[6].13 := SimulationDINT.21;
   			DataToSend[6].14 := SimulationDINT.22;
   			DataToSend[6].15 := SimulationDINT.23;
   			DataToSend[7].0  := SimulationDINT.8;
   			DataToSend[7].1  := SimulationDINT.9;
   			DataToSend[7].2  := SimulationDINT.10;
   			DataToSend[7].3  := SimulationDINT.11;
   			DataToSend[7].4  := SimulationDINT.12;
   			DataToSend[7].5  := SimulationDINT.13;
   			DataToSend[7].6  := SimulationDINT.14;
   			DataToSend[7].7  := SimulationDINT.15;
   			DataToSend[7].8  := SimulationDINT.0;
   			DataToSend[7].9  := SimulationDINT.1;
   			DataToSend[7].10 := SimulationDINT.2;
   			DataToSend[7].11 := SimulationDINT.3;
   			DataToSend[7].12 := SimulationDINT.4;
   			DataToSend[7].13 := SimulationDINT.5;
   			DataToSend[7].14 := SimulationDINT.6;
   			DataToSend[7].15 := SimulationDINT.7;
   
   			Trigger := TRUE;
   
   			if DeviceData.NewState then
   
   				DeviceData.StateDone := TRUE;
   
   			end_if;
   
   			if  DeviceData.CommSuccess and DeviceData.ReplayIndex = CMD_Index then
   
   				Trigger := FALSE;
   				DeviceData.OldState := DeviceData.State;
   				DeviceData.State := DeviceData.State + 1;
   				DeviceData.CommSuccess := FALSE;
   				DeviceData.AcyclicData[0] := 0;
   				DeviceData.NewState := TRUE;
   
   			 elsif DeviceData.CommTimeOut then
   
   				temp_string1 := 'Error in step ';
   				Temp_DINT := DeviceData.State;
   				DTOS(Temp_DINT, temp_string2);
   				CONCAT(temp_string1, temp_string2, qAOI_Diagnostic_String);
   
   				DeviceData.OldState := DeviceData.State;
   				DeviceData.State := DeviceData.MaxState;	//Check State
   				DeviceData.CommTimeOut := FALSE;
   				DeviceData.AcyclicData[0] := 0;
   				DeviceData.NewState := TRUE;
   
   			end_if;
   
   		//*********************************
   		21: // Totalizer 1 control
   		//*********************************
   
   			CMD_Index := 2100;
   			CMD_Subindex := 0;
   			CMD_Wr := TRUE;
   			CMD_Rd := FALSE;
   			CMD_ByteLength := 2;
   			DataToSend[6]:= 0;
   			DataToSend[7]:= 0;
   
   			DataToSend[6].9:= 1; // Preset + hold
   
   			Trigger := TRUE;
   
   			if DeviceData.NewState then
   
   				DeviceData.StateDone := TRUE;
   
   			end_if;
   
   			if  DeviceData.CommSuccess and DeviceData.ReplayIndex = CMD_Index then
   
   				Trigger := FALSE;
   				DeviceData.OldState := DeviceData.State;
   				DeviceData.State := DeviceData.MaxState;
   				DeviceData.CommSuccess := FALSE;
   				DeviceData.AcyclicData[0] := 0;
   				DeviceData.NewState := TRUE;
   
   			elsif DeviceData.CommTimeOut then
   
   				temp_string1 := 'Error in step ';
   				Temp_DINT := DeviceData.State;
   				DTOS(Temp_DINT, temp_string2);
   				CONCAT(temp_string1, temp_string2, qAOI_Diagnostic_String);
   
   				DeviceData.OldState := DeviceData.State;
   				DeviceData.State := DeviceData.MaxState;
   				DeviceData.CommTimeOut := FALSE;
   				DeviceData.AcyclicData[0] := 0;
   				DeviceData.NewState := TRUE;
   
   			end_if;
   
   
   		//***************************************
   	    30: // Read zero point adjustment status
   		//***************************************
   
   			CMD_Index := 8682;
   			CMD_Subindex := 0;
   			CMD_Wr := FALSE;
   			CMD_Rd := TRUE;
   			CMD_ByteLength := 2;
   			DataToSend[6]:= 0;
   			DataToSend[7]:= 0;
   			Trigger := TRUE;
   
   			if DeviceData.NewState then
   
   				DeviceData.StateDone := TRUE;
   
   			end_if;
   
   			if  DeviceData.CommSuccess and DeviceData.ReplayIndex = CMD_Index then
   
   				if DeviceData.AcyclicData[0] = 8 then
   
   					DeviceData.State := DeviceData.MaxState; // Zero Point already in progress
   					qAOI_Diagnostic_String := 'Zero point adjustement already in progress';
   
   				else
   
   					DeviceData.State := DeviceData.State + 1;
   
   				end_if;
   
   			Trigger := FALSE;
   			DeviceData.CommSuccess := FALSE;
   			DeviceData.AcyclicData[0] := 0;
   			DeviceData.NewState := TRUE;
   
   		elsif DeviceData.CommTimeOut then
   
   			temp_string1 := 'Error in step ';
   			Temp_DINT := DeviceData.State;
   			DTOS(Temp_DINT, temp_string2);
   			CONCAT(temp_string1, temp_string2, qAOI_Diagnostic_String);
   
   			DeviceData.OldState := DeviceData.State;
   			DeviceData.State := DeviceData.MaxState;
   			DeviceData.CommTimeOut := FALSE;
   			DeviceData.AcyclicData[0] := 0;
   			DeviceData.NewState := TRUE;
   
   		end_if;
   
   		//***************************************
   	    31: // Start zero point adjustment
   		//***************************************
   
   			CMD_Index := 8681;
   			CMD_Subindex := 0;
   			CMD_Wr := TRUE;	// Only Read or Write can be active
   			CMD_Rd := FALSE;
   			CMD_ByteLength := 2;	//Check Length
   			DataToSend[6] := 0;
   			DataToSend[7] := 0;
   			DataToSend[6].8 := 1;
   
   			Trigger := TRUE;
   
   			if DeviceData.NewState then
   
   				DeviceData.StateDone := TRUE;
   
   			end_if;
   
   			if  DeviceData.CommSuccess and DeviceData.ReplayIndex = CMD_Index then
   
   				Trigger := FALSE;
   				DeviceData.OldState := DeviceData.State;
   				DeviceData.State := DeviceData.State + 1;
   				DeviceData.CommSuccess := FALSE;
   				DeviceData.AcyclicData[0] := 0;
   				DeviceData.NewState := TRUE;
   
   			elsif DeviceData.CommTimeOut then
   
   				temp_string1 := 'Error in step ';
   				Temp_DINT := DeviceData.State;
   				DTOS(Temp_DINT, temp_string2);
   				CONCAT(temp_string1, temp_string2, qAOI_Diagnostic_String);
   
   				DeviceData.OldState := DeviceData.State;
   				DeviceData.State := DeviceData.MaxState;	//Check State
   				DeviceData.CommTimeOut := FALSE;
   				DeviceData.AcyclicData[0] := 0;
   				DeviceData.NewState := TRUE;
   
   			end_if;
   
   		//***************************************
   	    32: // Intermediate state
   		//***************************************
   			TONR (StandardTimer);
   			StandardTimer.PRE := 2000;
   			StandardTimer.TimerEnable := onlyonce;
   
   			CMD_Index := 297;
   			CMD_Subindex := 0;
   			CMD_Wr := FALSE;
   			CMD_Rd := TRUE;
   			CMD_ByteLength := 4;
   			DataToSend[6]:= 0;
   			DataToSend[7]:= 0;
   			Trigger := TRUE;
   
   			if DeviceData.NewState and not onlyonce then
   				DeviceData.StateDone := TRUE;
   			end_if;
   
   			if  DeviceData.CommSuccess and DeviceData.ReplayIndex = CMD_Index and not onlyonce then
   				Trigger := 0;
   				DeviceData.CommSuccess := FALSE;
   				DeviceData.AcyclicData[0] := 0;
   				DeviceData.NewState := TRUE;
   				onlyonce := TRUE;
   			end_if;
   
   			if StandardTimer.DN and onlyonce then
   				onlyonce := FALSE;
   				DeviceData.OldState := DeviceData.State;
   				DeviceData.State := DeviceData.State + 1;
   
   			end_if;
   
   
   		//***************************************
   	    33: // Read progress
   		//***************************************
   
   			CMD_Index := 2155;
   			CMD_Subindex := 0;
   			CMD_Wr := FALSE;
   			CMD_Rd := TRUE;
   			CMD_ByteLength := 2;
   			DataToSend[6]:= 0;
   			DataToSend[7]:= 0;
   			Trigger := TRUE;
   
   			if DeviceData.NewState then
   
   				DeviceData.StateDone := TRUE;
   
   			end_if;
   
   			if  DeviceData.CommSuccess and DeviceData.ReplayIndex = CMD_Index then
   
   				qReadProgress.0	:= DeviceData.AcyclicData[0].0;
   				qReadProgress.1	:= DeviceData.AcyclicData[0].1;
   				qReadProgress.2	:= DeviceData.AcyclicData[0].2;
   				qReadProgress.3	:= DeviceData.AcyclicData[0].3;
   				qReadProgress.4	:= DeviceData.AcyclicData[0].4;
   				qReadProgress.5	:= DeviceData.AcyclicData[0].5;
   				qReadProgress.6	:= DeviceData.AcyclicData[0].6;
   				qReadProgress.7	:= DeviceData.AcyclicData[0].7;
   
   				// Check if progress at 100 percent
   				if qReadProgress < 100 then
   
   					DeviceData.OldState := DeviceData.State - 2;
   					DeviceData.State := DeviceData.State - 1;
   					qZeroPointStatus := 8;
   
   				elsif qReadProgress = 100 then
   
   					DeviceData.OldState := DeviceData.State;
   					DeviceData.State := DeviceData.State + 1;
   
   				end_if;
   
   				Trigger := FALSE;
   				DeviceData.CommSuccess := FALSE;
   				DeviceData.AcyclicData[0] := 0;
   				DeviceData.NewState := TRUE;
   
   			elsif DeviceData.CommTimeOut then
   
   				temp_string1 := 'Error in step ';
   				Temp_DINT := DeviceData.State;
   				DTOS(Temp_DINT, temp_string2);
   				CONCAT(temp_string1, temp_string2, qAOI_Diagnostic_String);
   
   				DeviceData.OldState := DeviceData.State;
   				DeviceData.State := DeviceData.MaxState;
   				DeviceData.CommTimeOut := FALSE;
   				DeviceData.AcyclicData[0] := 0;
   				DeviceData.NewState := TRUE;
   
   			end_if;
   
   		//***************************************
   	    34: // Read zero point adjustment status
   		//***************************************
   
   			CMD_Index := 8682;
   			CMD_Subindex := 0;
   			CMD_Wr := 0;
   			CMD_Rd := TRUE;
   			CMD_ByteLength := 2;
   			DataToSend[6]:= 0;
   			DataToSend[7]:= 0;
   			Trigger := TRUE;
   
   			if DeviceData.NewState then
   
   				DeviceData.StateDone := TRUE;
   
   			end_if;
   
   			if  DeviceData.CommSuccess and DeviceData.ReplayIndex = CMD_Index then
   
   				qZeroPointStatus := DeviceData.AcyclicData[0];
   
   				if DeviceData.AcyclicData[0] = 8 then
   
   					qAOI_Diagnostic_String := 'Zero point adjustement already in progress';
   					DeviceData.OldState := DeviceData.State;
   					DeviceData.State := DeviceData.MaxState;
   
   				elsif DeviceData.AcyclicData[0] = 2 then
   
   					qAOI_Diagnostic_String := 'Zero point adjustement failed';
   					DeviceData.OldState := DeviceData.State;
   					DeviceData.State := DeviceData.MaxState;
   
   				elsif DeviceData.AcyclicData[0] = 5 then
   					qAOI_Diagnostic_String := 'Zero point adjustement done';
   					DeviceData.OldState := DeviceData.State;
   					DeviceData.State :=  DeviceData.MaxState;
   
   				end_if;
   
   				Trigger := FALSE;
   				DeviceData.CommSuccess := FALSE;
   				DeviceData.AcyclicData[0] := 0;
   				DeviceData.NewState := TRUE;
   
   			elsif DeviceData.CommTimeOut then
   
   				temp_string1 := 'Error in step ';
   				Temp_DINT := DeviceData.State;
   				DTOS(Temp_DINT, temp_string2);
   				CONCAT(temp_string1, temp_string2, qAOI_Diagnostic_String);
   
   				DeviceData.OldState := DeviceData.State;
   				DeviceData.State := DeviceData.MaxState;
   				DeviceData.CommTimeOut := FALSE;
   				DeviceData.AcyclicData[0] := 0;
   				DeviceData.NewState := TRUE;
   
   		end_if;
   
   		//*********************************
   		90: // Active diagnostic
   		//*********************************
   
   			CMD_Index := 297;
   			CMD_Subindex := 0;
   			CMD_Wr := FALSE;
   			CMD_Rd := TRUE;
   			CMD_ByteLength := 4;
   			DataToSend[6]:= 0;
   			DataToSend[7]:= 0;
   			Trigger := TRUE;
   
   			if DeviceData.NewState then
   				DeviceData.StateDone := TRUE;
   			end_if;
   
   			if  DeviceData.CommSuccess and DeviceData.ReplayIndex = CMD_Index then
   
   				qActual_Diagnostics_Code	:= DeviceData.AcyclicData[0];
   
   				case qActual_Diagnostics_Code of
   			        0:
   			            qActual_Diagnostics_String := '--------';
   			        16777312:
   			            qActual_Diagnostics_String := 'F437 Configuration incompatible';
   			        16777319:
   			            qActual_Diagnostics_String := 'F242 Firmware incompatible';
   			        16777323:
   			            qActual_Diagnostics_String := 'F252 Module incompatible';
   			        16777337:
   			            qActual_Diagnostics_String := 'F272 Electronic module faulty';
   			        16777340:
   			            qActual_Diagnostics_String := 'F270 Main electronics defective';
   			        16777341:
   			            qActual_Diagnostics_String := 'F271 Main electronics faulty';
   			        16777355:
   			            qActual_Diagnostics_String := 'F410 Data transfer failed';
   			        16777375:
   			            qActual_Diagnostics_String := 'F270 Main electronics defective';
   			        16777376:
   			            qActual_Diagnostics_String := 'F083 Memory content inconsistent';
   			        16777429:
   			            qActual_Diagnostics_String := 'F180 Temperature sensor defective';
   			        16777430:
   			            qActual_Diagnostics_String := 'F180 Temperature sensor defective';
   			        16777441:
   			            qActual_Diagnostics_String := 'F283 Memory content inconsistent';
   			        16777445:
   			            qActual_Diagnostics_String := 'F273 Main electronics defective';
   			        16777447:
   			            qActual_Diagnostics_String := 'F082 Data storage inconsistent';
   			        16777499:
   			            qActual_Diagnostics_String := 'F938 Coil current not stable';
   			        16777500:
   			            qActual_Diagnostics_String := 'F181 Sensor connection faulty';
   			        16777547:
   			            qActual_Diagnostics_String := 'F201 Electronics faulty';
   			        16777583:
   			            qActual_Diagnostics_String := 'F283 Memory content inconsistent';
   			        16777930:
   			            qActual_Diagnostics_String := 'F331 Firmware update failed in module 1';
   			        16778490:
   			            qActual_Diagnostics_String := 'F419 Power cycle required';
   			        16843466:
   			            qActual_Diagnostics_String := 'F331 Firmware update failed in module 2';
   			        33554573:
   			            qActual_Diagnostics_String := 'C492 Frequency output simulation active';
   			        33554574:
   			            qActual_Diagnostics_String := 'C493 Pulse output simulation active';
   			        33554575:
   			            qActual_Diagnostics_String := 'C494 Switch output simulation active';
   			        33554576:
   			            qActual_Diagnostics_String := 'C484 Failure mode simulation active';
   			        33554579:
   			            qActual_Diagnostics_String := 'C485 Process variable simulation active';
   			        33554580:
   			            qActual_Diagnostics_String := 'C453 Flow override active';
   			        33554782:
   			            qActual_Diagnostics_String := 'C495 Diagnostic event simulation active';
   			        33554948:
   			            qActual_Diagnostics_String := 'C412 Processing download';
   			        67108970:
   			            qActual_Diagnostics_String := 'M438 Dataset different';
   			        67109090:
   			            qActual_Diagnostics_String := 'M311 Electronic module faulty';
   			        134217866:
   			            qActual_Diagnostics_String := 'S442 Frequency output saturated';
   			        134217868:
   			            qActual_Diagnostics_String := 'S443 Pulse output saturated';
   			        134217873:
   			            qActual_Diagnostics_String := 'S842 Process value below limit';
   			        134217925:
   			            qActual_Diagnostics_String := 'S834 Process temperature too high';
   			        134217926:
   			            qActual_Diagnostics_String := 'S835 Process temperature too low';
   			        134218013:
   			            qActual_Diagnostics_String := 'S004 Sensor defective';
   			        134218017:
   			            qActual_Diagnostics_String := 'S443 Pulse output saturated';
   			        134218018:
   			            qActual_Diagnostics_String := 'S442 Frequency output saturated';
   			        134218068:
   			            qActual_Diagnostics_String := 'S937 Sensor symmetry';
   			        134218069:
   			            qActual_Diagnostics_String := 'S961 Electrode potential out of specification';
   			        134219072:
   			            qActual_Diagnostics_String := 'S880 Output overloaded';
   			        134219092:
   			            qActual_Diagnostics_String := 'S004 Sensor defective';
   
   				else
   
   					qActual_Diagnostics_String := 'Error Code unknown';
   
   				end_case;
   
   				Trigger := 0;
   				DeviceData.OldState := DeviceData.State;
   		        DeviceData.State := DeviceData.State + 1;
   				DeviceData.CommSuccess := FALSE;
   				DeviceData.AcyclicData[0] := 0;
   				DeviceData.NewState := TRUE;
   
   
   			 elsif DeviceData.CommTimeOut then
   
   				temp_string1 := 'Error in step ';
   				Temp_DINT := DeviceData.State;
   				DTOS(Temp_DINT, temp_string2);
   				CONCAT(temp_string1, temp_string2, qAOI_Diagnostic_String);
   
   				DeviceData.OldState := DeviceData.State;
   				DeviceData.State := DeviceData.MaxState;	//Check State
   				DeviceData.CommTimeOut := FALSE;
   				DeviceData.AcyclicData[0] := 0;
   				DeviceData.NewState := TRUE;
   
   		    end_if;
   
   		//*********************************
   	    91: // Previous Diagnostic
   	    //*********************************
   
   		    CMD_Index := 298;
   			CMD_Subindex := 0;
   		    CMD_Wr := FALSE;
   			CMD_Rd := TRUE;
   			CMD_ByteLength := 4;
   			DataToSend[6]:= 0;
   			DataToSend[7]:= 0;
   			Trigger := TRUE;
   
   			if DeviceData.NewState then
   				DeviceData.StateDone := TRUE;
   			end_if;
   
   			if  DeviceData.CommSuccess and DeviceData.ReplayIndex = CMD_Index then
   
   				qLast_Diagnostics_Code	:= DeviceData.AcyclicData[0];
   
   				case qLast_Diagnostics_Code of
   			        0:
   			            qLast_Diagnostics_String := '--------';
   			        16777312:
   			            qLast_Diagnostics_String := 'F437 Configuration incompatible';
   			        16777319:
   			            qLast_Diagnostics_String := 'F242 Firmware incompatible';
   			        16777323:
   			            qLast_Diagnostics_String := 'F252 Module incompatible';
   			        16777337:
   			            qLast_Diagnostics_String := 'F272 Electronic module faulty';
   			        16777340:
   			            qLast_Diagnostics_String := 'F270 Main electronics defective';
   			        16777341:
   			            qLast_Diagnostics_String := 'F271 Main electronics faulty';
   			        16777355:
   			            qLast_Diagnostics_String := 'F410 Data transfer failed';
   			        16777375:
   			            qLast_Diagnostics_String := 'F270 Main electronics defective';
   			        16777376:
   			            qLast_Diagnostics_String := 'F083 Memory content inconsistent';
   			        16777429:
   			            qLast_Diagnostics_String := 'F180 Temperature sensor defective';
   			        16777430:
   			            qLast_Diagnostics_String := 'F180 Temperature sensor defective';
   			        16777441:
   			            qLast_Diagnostics_String := 'F283 Memory content inconsistent';
   			        16777445:
   			            qLast_Diagnostics_String := 'F273 Main electronics defective';
   			        16777447:
   			            qLast_Diagnostics_String := 'F082 Data storage inconsistent';
   			        16777499:
   			            qLast_Diagnostics_String := 'F938 Coil current not stable';
   			        16777500:
   			            qLast_Diagnostics_String := 'F181 Sensor connection faulty';
   			        16777547:
   			            qLast_Diagnostics_String := 'F201 Electronics faulty';
   			        16777583:
   			            qLast_Diagnostics_String := 'F283 Memory content inconsistent';
   			        16777930:
   			            qLast_Diagnostics_String := 'F331 Firmware update failed in module 1';
   			        16778490:
   			            qLast_Diagnostics_String := 'F419 Power cycle required';
   			        16843466:
   			            qLast_Diagnostics_String := 'F331 Firmware update failed in module 2';
   			        33554573:
   			            qLast_Diagnostics_String := 'C492 Frequency output simulation active';
   			        33554574:
   			            qLast_Diagnostics_String := 'C493 Pulse output simulation active';
   			        33554575:
   			            qLast_Diagnostics_String := 'C494 Switch output simulation active';
   			        33554576:
   			            qLast_Diagnostics_String := 'C484 Failure mode simulation active';
   			        33554579:
   			            qLast_Diagnostics_String := 'C485 Process variable simulation active';
   			        33554580:
   			            qLast_Diagnostics_String := 'C453 Flow override active';
   			        33554782:
   			            qLast_Diagnostics_String := 'C495 Diagnostic event simulation active';
   			        33554948:
   			            qLast_Diagnostics_String := 'C412 Processing download';
   			        67108970:
   			            qLast_Diagnostics_String := 'M438 Dataset different';
   			        67109090:
   			            qLast_Diagnostics_String := 'M311 Electronic module faulty';
   			        134217866:
   			            qLast_Diagnostics_String := 'S442 Frequency output saturated';
   			        134217868:
   			            qLast_Diagnostics_String := 'S443 Pulse output saturated';
   			        134217873:
   			            qLast_Diagnostics_String := 'S842 Process value below limit';
   			        134217925:
   			            qLast_Diagnostics_String := 'S834 Process temperature too high';
   			        134217926:
   			            qLast_Diagnostics_String := 'S835 Process temperature too low';
   			        134218013:
   			            qLast_Diagnostics_String := 'S004 Sensor defective';
   			        134218017:
   			            qLast_Diagnostics_String := 'S443 Pulse output saturated';
   			        134218018:
   			            qLast_Diagnostics_String := 'S442 Frequency output saturated';
   			        134218068:
   			            qLast_Diagnostics_String := 'S937 Sensor symmetry';
   			        134218069:
   			            qLast_Diagnostics_String := 'S961 Electrode potential out of specification';
   			        134219072:
   			            qLast_Diagnostics_String := 'S880 Output overloaded';
   			        134219092:
   			            qLast_Diagnostics_String := 'S004 Sensor defective';
   				else
   					qLast_Diagnostics_String := 'Error Code unknown';
   
   				end_case;
   
   				Trigger := FALSE;
   				DeviceData.OldState := DeviceData.State;
   		        DeviceData.State := DeviceData.MaxState;
   				DeviceData.CommSuccess := FALSE;
   				DeviceData.AcyclicData[0] := 0;
   				DeviceData.NewState := TRUE;
   
   			 elsif DeviceData.CommTimeOut then
   
   				temp_string1 := 'Error in step ';
   				Temp_DINT := DeviceData.State;
   				DTOS(Temp_DINT, temp_string2);
   				CONCAT(temp_string1, temp_string2, qAOI_Diagnostic_String);
   
   				DeviceData.OldState := DeviceData.State;
   				DeviceData.State := DeviceData.MaxState;	//Check State
   				DeviceData.CommTimeOut := FALSE;
   				DeviceData.AcyclicData[0] := 0;
   				DeviceData.NewState := TRUE;
   
   			end_if;
   
   		//*********************************
   		98: // End Step Trigger Guard
   		//*********************************
   
   				DeviceData.State := 0;
   				CommAOIBusy := 0;
   				DeviceAOISendRequest.[DeviceData.DevicePort] := FALSE;
   				ActiveComPort := 0;
   				ActiveAOI := FALSE;
   				DataToSend[0] := 0;
   				DataToSend[1] := 0;
   				DataToSend[2] := 0;
   				DataToSend[3] := 0;
   				DataToSend[4] := 0;
   				DataToSend[5] := 0;
    				DataToSend[6] := 0;
   				DataToSend[7] := 0;
    				DataToSend[8] := 0;
   				DataToSend[9] := 0;
   				DeviceData.StateDone := FALSE;
   				Skip := FALSE;
   				DeviceData.State := 0;
   				firstTimeDone := FALSE;
   				DeviceData.NewState := FALSE;
   				DeviceData.OldState := 0;
   				ActiveAOI := FALSE;
   
   				if PulseSimActive then
   
   					PulseSimActive := FALSE;
   					PulseSimChanged := FALSE;
   
   				elsif TotActive then
   
   					TotActive := FALSE;
   					TotChanged := FALSE;
   
   				elsif ZeroPointActive then
   
   					ZeroPointActive := FALSE;
   					StartZeroPointAdjustmentChanged := FALSE;
   
   				elsif ParameterizeActive then
   
   					ParameterizeActive := FALSE;
   					ParameterizeChanged := FALSE;
   
   				elsif CondStatusActive then
   
   					CondStatusActive := FALSE;
   					CondStatusChanged := FALSE;
   
   				end_if;
   
   	end_case;
   
   	end_if;
   
   	//*************************
   	// Execution Area
   	//*************************
   	if DeviceData.State > StateMin and DeviceData.State < DeviceData.MaxState then
   
   		DataToSend[2] := DeviceData.DevicePort;
   		DataToSend[3] := CMD_Index;
   		DataToSend[4] := CMD_Subindex;
   		DataToSend[5].0 := CMD_Rd;
   		DataToSend[5].1 := CMD_Wr;
   		DataToSend[5].8 := CMD_ByteLength.0;  // Bits for the Length of the Data
   		DataToSend[5].9 := CMD_ByteLength.1;
   		DataToSend[5].10 := CMD_ByteLength.2;
   		DataToSend[5].11 := CMD_ByteLength.3;
   		DataToSend[5].12 := CMD_ByteLength.4;
   		DataToSend[5].13 := CMD_ByteLength.5;
   		DataToSend[5].14 := CMD_ByteLength.6;
   		DataToSend[5].15 := CMD_ByteLength.7;
   		DataToSend[5].7 := Trigger;
   
   		qCommError := CommError;
   
   	end_if;
   
   
   end_if;
END_ROUTINE
END_ADD_ON_INSTRUCTION
